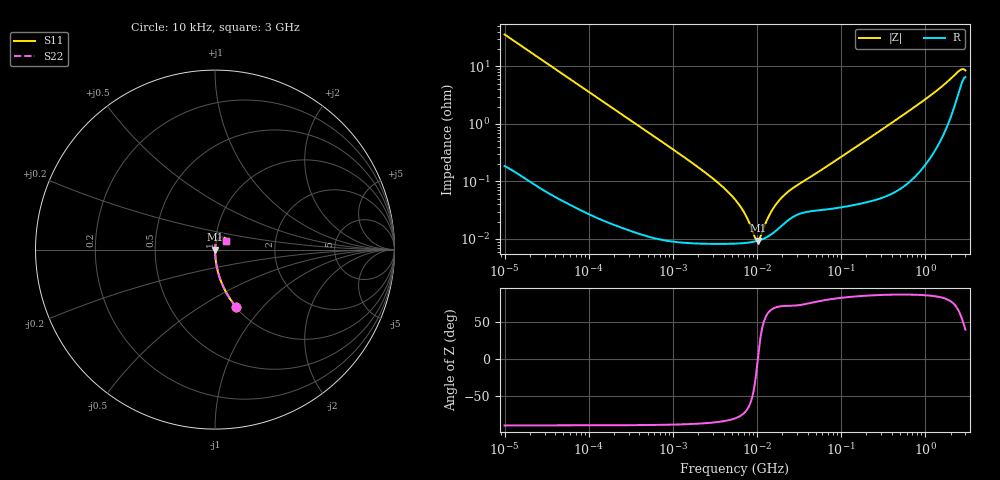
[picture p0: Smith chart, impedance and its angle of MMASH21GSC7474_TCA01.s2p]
! MMASH21GSC7474_TCA01  S-PARAMETER MODEL  ( Standard Model )
! Model Generated by TAIYO YUDEN Corporation (http://www.ty-top.com)
! Version 1.0
! TAIYO YUDEN Control No. 220601
! Copyright(c) 2016 TAIYO YUDEN CO.,LTD. All Rights Reserved.
! Product Description (link to TY-COMPAS)
! https://ds.yuden.co.jp/TYCOMPAS/or/detail?pn=MMASH21GSC7474KTCA01&u=M
! Products Name : Multilayer Ceramic Capacitors
! Characteristics :
!  Capacitance : 0.47 [uF] , Rated Voltage : 100 [V] , TCC : X7S
!  Case Size : 2.0 x 1.25 / 0.079 x 0.049 [mm/inch] , Thickness : 1.25 / 0.049 [mm/inch]
!  (Conditions: Temperature = 25 [degC] , DC Bias Voltage = 0 [V])
! External Node Assignments :
!  1  o---| |---o  2
! GND o---------o GND
! Frequency Range : 10kHz  -  3GHz  [ 401 STEP ]
# MHZ S RI R 50
! Freq[MHz].  S11 Real  S11 Imag  S21 Real  S21 Imag  S12 Real  S12 Imag  S22 Real  S22 Imag
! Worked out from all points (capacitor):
!   401 points, 10 kHz to 3 GHz, reference 50 ohm
!   read as one part in series: C = 441 nF near 10.65 kHz
!   lowest |Z| = 9.33 mohm at 10.29 MHz (marker M1)
!   series resonance near 10.22 MHz, so ESL is about 550 pH
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0.01  0.1161 -0.3178  0.8839 0.3178  0.8839 0.3178  0.1161 -0.3178
0.015549  0.0522 -0.2197  0.9478 0.2197  0.9478 0.2197  0.0522 -0.2197
0.026575  0.0189 -0.1334  0.9811 0.1334  0.9811 0.1334  0.0189 -0.1334
0.082683  0.00223 -0.0438  0.9978 0.0438  0.9978 0.0438  0.00223 -0.0438
0.683653  0.000127 -0.00532  0.9999 0.00532  0.9999 0.00532  0.000127 -0.00532
2.737278  8.36e-05 -0.00124  0.9999 0.00124  0.9999 0.00124  8.36e-05 -0.00124
4.124064  8.25e-05 -0.000746  0.9999 0.000746  0.9999 0.000746  8.25e-05 -0.000746
5.477226  8.3e-05 -0.000479  0.9999 0.000479  0.9999 0.000479  8.3e-05 -0.000479
7.274378  8.51e-05 -0.000251  0.9999 0.000251  0.9999 0.000251  8.51e-05 -0.000251
9.361346  9e-05 -6.4e-05  0.9999 6.4e-05  0.9999 6.4e-05  9e-05 -6.4e-05
10.29003  9.32e-05 4.85e-06  0.9999 -4.85e-06  0.9999 -4.85e-06  9.32e-05 4.85e-06
11.31085  9.75e-05 7.39e-05  0.9999 -7.39e-05  0.9999 -7.39e-05  9.75e-05 7.39e-05
12.83117  0.000106 0.000167  0.9999 -0.000167  0.9999 -0.000167  0.000106 0.000167
14.55585  0.000118 0.000262  0.9999 -0.000262  0.9999 -0.000262  0.000118 0.000262
18.73182  0.000159 0.000457  0.9998 -0.000457  0.9998 -0.000457  0.000159 0.000457
25.67485  0.000232 0.000697  0.9998 -0.000697  0.9998 -0.000697  0.000232 0.000697
45.28751  0.000307 0.00121  0.9997 -0.00121  0.9997 -0.00121  0.000307 0.00121
374.4521  0.000678 0.00977  0.9993 -0.00977  0.9993 -0.00977  0.000678 0.00977
1202.347  0.00389 0.0325  0.9961 -0.0325  0.9961 -0.0325  0.00389 0.0325
2482.93  0.0381 0.0695  0.9619 -0.0695  0.9619 -0.0695  0.0381 0.0695
2729.247  0.0543 0.0653  0.9457 -0.0653  0.9457 -0.0653  0.0543 0.0653
3000  0.064 0.0477  0.936 -0.0477  0.936 -0.0477  0.064 0.0477
